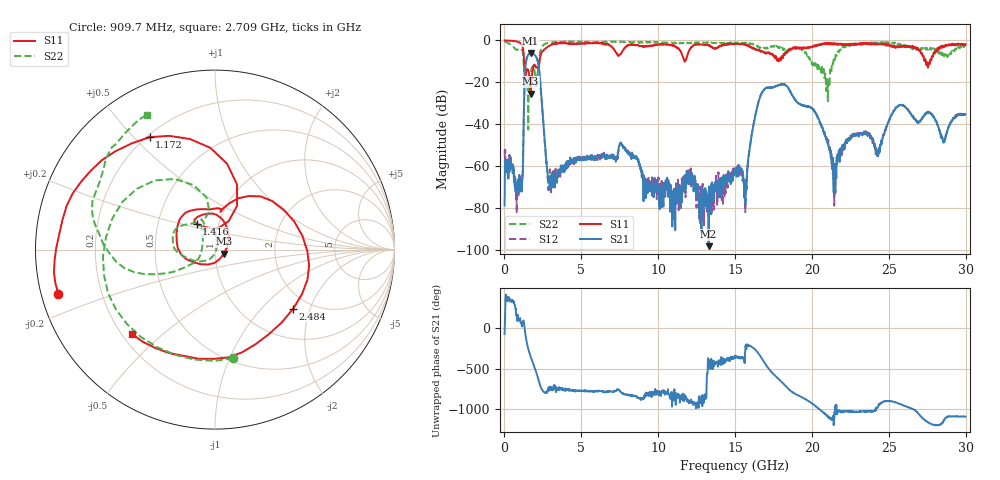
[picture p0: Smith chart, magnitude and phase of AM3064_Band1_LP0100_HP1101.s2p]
# Hz S DB R 50.0
!freq dBS11 angS11 dBS21 angS21 dBS12 angS12 dBS22 angS22
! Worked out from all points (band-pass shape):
!   1600 points, 10 MHz to 29.98 GHz, reference 50 ohm
!   highest |S21| = -6.02 dB at 1.697 GHz (marker M1); lowest = -98.1 dB at 13.28 GHz (marker M2)
!   |S21| within 3 dB of the highest: 1.435 GHz to 2.13 GHz (694.8 MHz wide, 39 % of centre)
!   lowest |S11| = -25.4 dB at 1.697 GHz (marker M3), VSWR 1.11, Z = 55.1 - j2.53 ohm
!   |S11| at or under -10 dB: 1.277 GHz to 2.28 GHz (1.003 GHz wide, 56.4 % of centre); 11.70454 GHz to 11.75281 GHz (48.27 MHz wide, 0.412 % of centre); 27.4 GHz to 27.68 GHz (281.1 MHz wide, 1.02 % of centre)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
!   |S22| runs from -42.5 to -0.4 dB; largest |S21 - S12| = 0.0089
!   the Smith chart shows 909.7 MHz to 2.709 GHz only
!   S11 on the Smith chart (normalised r, x): 909.7 MHz: 0.05, -0.14; 1.172 GHz: 0.21, +0.56; 1.416 GHz: 0.78, +0.23; 2.484 GHz: 1.64, -1.54; 2.709 GHz: 0.24, -0.40
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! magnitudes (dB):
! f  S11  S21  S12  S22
! 10 MHz  -0.1  -78.7  -52.4  -0.4
! 909.7 MHz  -0.9  -67.4  -74.5  -4.2
! 1.172 GHz  -2.8  -66.1  -64.6  -5.2
! 1.416 GHz  -15.1  -9.7  -9.6  -18.7
! 1.697 GHz  -25.4  -6.0  -6.0  -15.8
! 2.166 GHz  -13.2  -10.0  -9.9  -15.0
! 2.484 GHz  -5.3  -34.7  -34.6  -2.6
! 2.709 GHz  -3.6  -56.2  -56.8  -1.5
! 3.009 GHz  -2.2  -66.8  -67.9  -1.0
! 5.015 GHz  -1.5  -56.6  -55.6  -0.8
! 7.657 GHz  -5.3  -49.9  -50.2  -0.7
! 10 GHz  -2.0  -69.4  -68.1  -1.0
! 13.28 GHz  -2.5  -98.1  -84.0  -1.2
! 15 GHz  -1.7  -62.0  -61.6  -1.4
! 15.7 GHz  -2.2  -67.8  -79.3  -1.3
! 16.95 GHz  -5.8  -23.0  -23.0  -3.6
! 19.99 GHz  -3.4  -32.4  -32.5  -10.9
! 21.02 GHz  -1.3  -48.9  -48.3  -26.6
! 21.45 GHz  -2.0  -63.7  -78.8  -8.5
! 25 GHz  -2.0  -38.4  -38.4  -1.2
! 28.54 GHz  -2.5  -48.3  -48.6  -6.2
! 29.98 GHz  -1.9  -35.4  -35.5  -2.8
